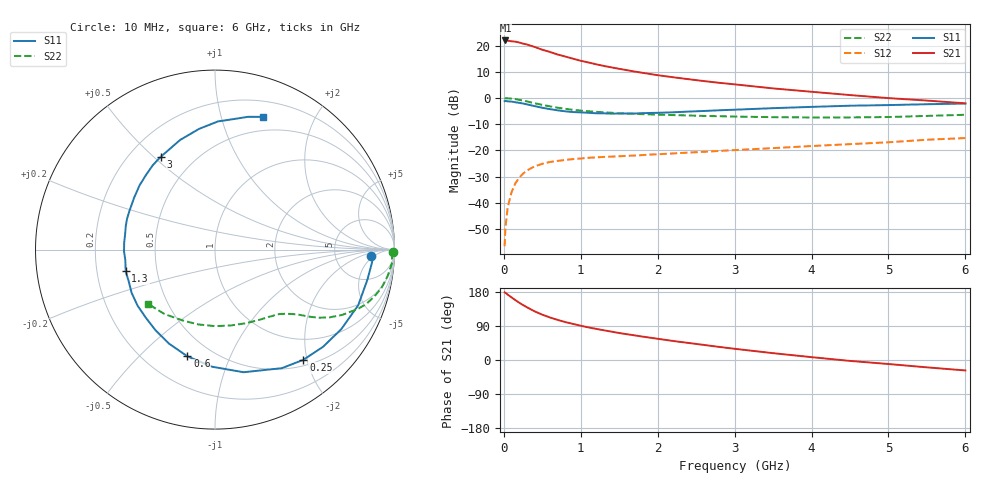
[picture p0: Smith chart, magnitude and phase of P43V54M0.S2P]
! SIEMENS Small Signal Semiconductors
! BFP182
! Si NPN RF Bipolar Junction Transistor in SOT143
! VCE = 3.5 V  IC = 4 mA
! Common Emitter S-Parameters:  March  1996
# GHz  S  MA  R  50
!  f  S11  S21  S12  S22
! GHz  MAG  ANG  MAG  ANG  MAG  ANG  MAG  ANG
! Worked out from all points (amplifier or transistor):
!   36 points, 10 MHz to 6 GHz, reference 50 ohm
!   highest |S21| = 22.0 dB at 20 MHz (marker M1)
!   |S21| within 3 dB of that: start of sweep to 449.4 MHz
!   unconditionally stable (mu >= 1): 1.713 GHz to 5.579 GHz
!   at 250 MHz: K = 0.18, MSG = 24.8 dB, |S12| = -28.8 dB
!   at 1.4 GHz: K = 0.87, MSG = 17.0 dB, |S12| = -22.3 dB
!   at 6 GHz: K = 0.94, MSG = 6.6 dB, |S12| = -15.3 dB
!   S11 on the Smith chart (normalised r, x): 10 MHz: 14, -4; 250 MHz: 0.60, -1.93; 600 MHz: 0.37, -0.71; 1.3 GHz: 0.33, -0.11; 3 GHz: 0.33, +0.53; 6 GHz: 0.35, +1.36
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0.01  0.8723 -2.2  12.34 178.6  0.0015 88.6  0.9924 -0.9
0.02  0.8784 -4.4  12.53 177.4  0.0033 87.3  0.9875 -1.8
0.05  0.866 -10.9  12.43 172.5  0.0083 87.8  0.9887 -4.4
0.15  0.8316 -32.2  11.88 158.0  0.0237 72.5  0.9527 -12.8
0.2  0.8097 -42.0  11.45 151.2  0.0303 67.8  0.9254 -16.4
0.25  0.787 -51.3  10.9 144.9  0.0363 63.0  0.8956 -19.8
0.3  0.7583 -60.6  10.51 139.2  0.0416 58.6  0.8616 -22.6
0.4  0.7015 -76.9  9.416 128.4  0.0498 52.1  0.7964 -27.2
0.5  0.6526 -91.5  8.341 119.6  0.0558 46.1  0.7416 -30.6
0.6  0.6141 -104.5  7.559 112.2  0.0605 41.9  0.6947 -33.1
0.7  0.5829 -116.2  6.759 105.8  0.0634 38.8  0.654 -35.0
0.8  0.5584 -126.4  6.178 100.0  0.0661 36.4  0.6218 -36.4
1  0.5326 -144.1  5.129 90.4  0.0704 32.9  0.5766 -38.7
1.1  0.5233 -152.6  4.765 86.0  0.0726 31.8  0.5595 -39.9
1.3  0.5119 -166.4  4.093 78.4  0.0754 30.2  0.5341 -42.0
1.6  0.5075 175.5  3.399 68.0  0.0791 29.1  0.5053 -45.4
2.2  0.5349 147.6  2.492 50.2  0.0879 28.5  0.4732 -53.6
3  0.5993 120.2  1.824 29.6  0.1018 27.7  0.4437 -67.8
3.5  0.6412 107.6  1.527 18.0  0.111 26.5  0.4318 -78.3
4.5  0.7142 88.7  1.14 -2.4  0.1322 23.2  0.4271 -102.5
5.5  0.7625 76.0  0.895 -19.4  0.1605 19.0  0.4565 -128.3
6  0.7855 70.3  0.793 -27.6  0.1727 14.9  0.4799 -140.9
